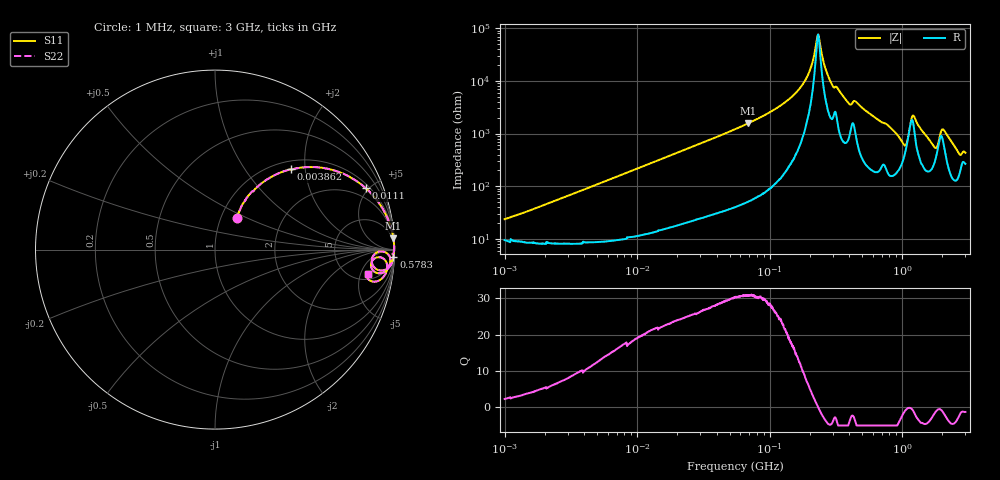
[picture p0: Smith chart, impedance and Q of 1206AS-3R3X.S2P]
!s-Parameter Generated by FASTRON Sdn. Bhd.
!FASTRON P/N : 1206AS-3R3X
!Keysight Technologies: E4991B_MY54100416_A.01.15
!Date created: Thu Nov 16 13:54:14 2023
!Version  : Rev00 Thu Nov 16 13:54:14 2023
!Data & Calibration Information:
!Freq	S11	S21	S12	S22
!PortZ  Port1:50+j0  Port2:50+j0
!When reading reference impedance value at option line is always used.
! Remarks : This data is being provided solely for informational purposes.
# Hz S dB R 50
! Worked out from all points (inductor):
!   1601 points, 1 MHz to 3 GHz, reference 50 ohm
!   read as one part in series: L = 3.45 uH near 1.24 MHz
!   highest Q = 30.9 at 68.95 MHz (marker M1), where L = 3.62 uH
!   self-resonance near 231.4 MHz
!   S11 on the Smith chart (normalised r, x): 1 MHz: 1.19, +0.43; 3.862 MHz: 1.16, +1.67; 11.1 MHz: 1.24, +4.78; 578.3 MHz: 5, -46; 3 GHz: 6.32, -6.80
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1000000  -13.46 55.2  -0.95 -11.2  -0.95 -11.2  -13.46 55.2
3804036  -4.31 47.1  -2.67 -37.3  -2.67 -37.3  -4.31 47.1
3861573  -4.23 46.7  -2.72 -37.7  -2.72 -37.7  -4.23 46.7
1.109966e7  -0.85 22.2  -8.43 -64.9  -8.43 -64.9  -0.85 22.2
1.447069e7  -0.54 17.5  -10.41 -69.8  -10.41 -69.8  -0.54 17.5
5.477226e7  -0.05 4.7  -21.70 -83.4  -21.70 -83.4  -0.05 4.7
6.894898e7  -0.04 3.6  -23.95 -84.5  -23.95 -84.5  -0.04 3.6
1.49005e8  -0.01 1.1  -34.29 -85.5  -34.29 -85.5  -0.01 1.1
1.829372e8  -0.01 0.6  -39.74 -83.1  -39.74 -83.1  -0.01 0.6
2.083556e8  -0.01 0.3  -46.34 -75.0  -46.34 -75.0  -0.01 0.3
2.3377e8  -0.01 -0.0  -57.31 11.7  -57.31 11.7  -0.01 -0.0
2.622844e8  -0.01 -0.3  -45.03 73.8  -45.03 73.8  -0.01 -0.3
2.972367e8  -0.02 -0.7  -38.36 76.1  -38.36 76.1  -0.02 -0.7
3.953438e8  -0.05 -1.5  -31.53 76.0  -31.53 76.0  -0.05 -1.5
5.7828e8  -0.04 -2.5  -27.35 82.4  -27.35 82.4  -0.04 -2.5
7.925923e8  -0.10 -4.0  -22.96 79.1  -22.96 79.1  -0.10 -4.0
1.0437e9  -0.97 -6.5  -16.47 42.2  -16.47 42.2  -0.97 -6.5
1.218836e9  -0.26 -1.9  -27.07 46.7  -27.07 46.7  -0.26 -1.9
1.738771e9  -0.77 -8.2  -15.84 54.2  -15.84 54.2  -0.77 -8.2
2.040726e9  -0.43 -3.7  -21.99 51.1  -21.99 51.1  -0.43 -3.7
2.660507e9  -0.84 -11.4  -13.56 58.4  -13.56 58.4  -0.84 -11.4
3e9  -1.27 -9.1  -13.98 42.9  -13.98 42.9  -1.27 -9.1
